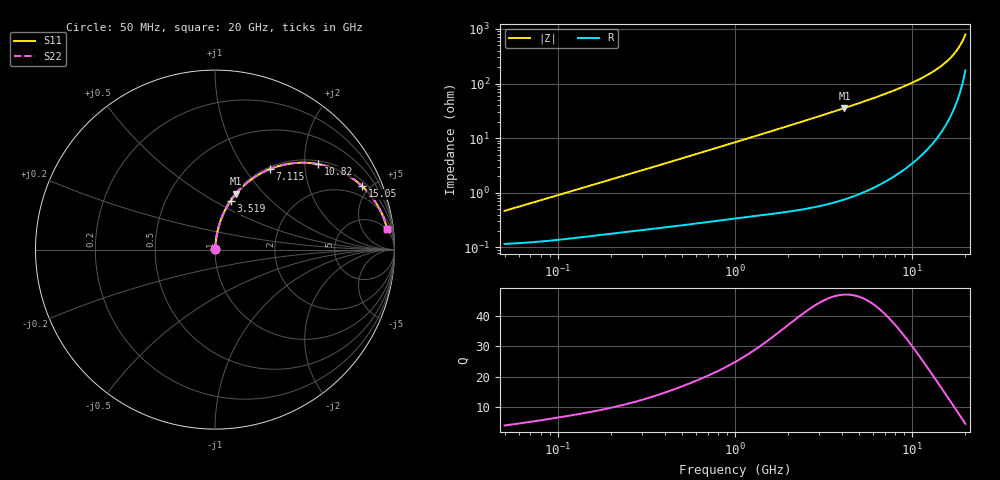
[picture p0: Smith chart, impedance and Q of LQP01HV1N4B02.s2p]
!Murata Part Number: LQP01HV1N4B02
!These Parameters are Measured in Series Mode Connection
!  o--[Z]--o
!Port1  Port2
!  o-------o
!Freq. Start=50[MHz] Stop=20[GHz], 401[Steps]
# Hz S RI R 50
!Freq.(Hz) S11(Real) S11(Imag) S21(Real) S21(Imag) S12(Real) S12(Imag) S22(Real) S22(Imag)
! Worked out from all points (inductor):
!   401 points, 50 MHz to 20 GHz, reference 50 ohm
!   read as one part in series: L = 1.44 nH near 51.52 MHz
!   highest Q = 47 at 4.149 GHz (marker M1), where L = 1.36 nH
!   S11 on the Smith chart (normalised r, x): 50 MHz: 1.00, +0.01; 3.519 GHz: 1.01, +0.60; 7.115 GHz: 1.03, +1.31; 10.82 GHz: 1.09, +2.33; 15.05 GHz: 1.30, +4.51; 20 GHz: 4, +15
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5e7  0.00118 0.00452  0.9988 -0.00452  0.9988 -0.00452  0.00118 0.00452
1.364002e8  0.00168 0.012  0.9983 -0.012  0.9983 -0.012  0.00168 0.012
3.721004e8  0.00326 0.0317  0.9967 -0.0317  0.9967 -0.0317  0.00326 0.0317
6.380365e8  0.00567 0.0535  0.9943 -0.0535  0.9943 -0.0535  0.00567 0.0535
1e9  0.0103 0.0828  0.9897 -0.0828  0.9897 -0.0828  0.0103 0.0828
1.689197e9  0.0235 0.1374  0.9765 -0.1374  0.9765 -0.1374  0.0235 0.1374
2.728004e9  0.0546 0.2158  0.9454 -0.2158  0.9454 -0.2158  0.0546 0.2158
3.519108e9  0.0868 0.271  0.9132 -0.271  0.9132 -0.271  0.0868 0.271
4.149438e9  0.1174 0.3114  0.8826 -0.3114  0.8826 -0.3114  0.1174 0.3114
5.515528e9  0.1961 0.3861  0.8039 -0.3861  0.8039 -0.3861  0.1961 0.3861
7.114996e9  0.3041 0.4478  0.6959 -0.4478  0.6959 -0.4478  0.3041 0.4478
7.442007e9  0.3276 0.4567  0.6724 -0.4567  0.6724 -0.4567  0.3276 0.4567
9.178299e9  0.4551 0.483  0.5449 -0.483  0.5449 -0.483  0.4551 0.483
1.082228e10  0.5735 0.4766  0.4265 -0.4766  0.4265 -0.4766  0.5735 0.4766
1.295331e10  0.7114 0.4297  0.2886 -0.4297  0.2886 -0.4297  0.7114 0.4297
1.396067e10  0.7676 0.3956  0.2324 -0.3956  0.2324 -0.3956  0.7676 0.3956
1.504638e10  0.8205 0.3523  0.1795 -0.3523  0.1795 -0.3523  0.8205 0.3523
1.621653e10  0.8683 0.3003  0.1317 -0.3003  0.1317 -0.3003  0.8683 0.3003
1.747767e10  0.9091 0.24  0.0909 -0.24  0.0909 -0.24  0.9091 0.24
1.855685e10  0.9354 0.1868  0.0646 -0.1868  0.0646 -0.1868  0.9354 0.1868
1.940974e10  0.9509 0.1444  0.0491 -0.1444  0.0491 -0.1444  0.9509 0.1444
2e10  0.959 0.1153  0.041 -0.1153  0.041 -0.1153  0.959 0.1153
